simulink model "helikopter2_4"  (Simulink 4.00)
settings: Solver=ode1  SolverMode=SingleTasking  StartTime=0.0  StopTime=999999  FixedStep=0.005  MaxStep=10  RelTol=1e-3  AbsTol=1e-3
undefined symbols (not defined in the file or in its folder): simget
libraries: qctools x7

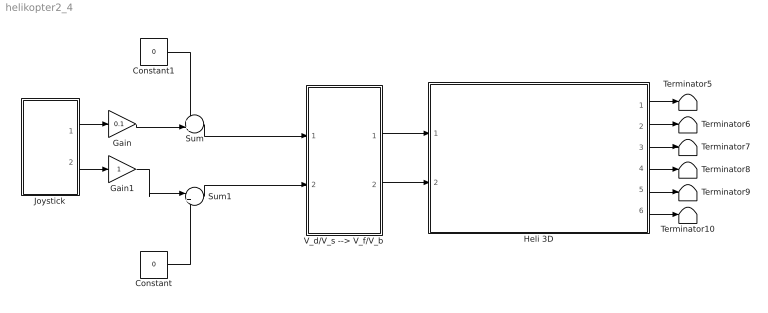
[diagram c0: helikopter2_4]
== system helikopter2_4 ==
  Constant : Constant  Value=0
  Constant1 : Constant  Value=0
  Gain : Gain  Gain=0.1  Multiplication=Element-wise(K.*u)  SaturateOnIntegerOverflow=on
  Gain1 : Gain  Gain=1  Multiplication=Element-wise(K.*u)  SaturateOnIntegerOverflow=on
  Heli 3D : Subsystem
  Joystick : Subsystem
  Sum : Sum  Inputs=++|  SaturateOnIntegerOverflow=on
  Sum1 : Sum  Inputs=|++  SaturateOnIntegerOverflow=on
  Terminator{5..10} (6 alike) : Terminator
  V_d/V_s --> V_f/V_b : Subsystem
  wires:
  V_d/V_s --> V_f/V_b/2(V_b) -> Heli 3D/2("V_b, motor bak")
  V_d/V_s --> V_f/V_b/1(V_f) -> Heli 3D/1("V_f, motor foran")
  Heli 3D/1("Vandring, (grader)") -> Terminator5/1
  Heli 3D/2("Vandringsrate, (grader/sek)") -> Terminator6/1
  Heli 3D/3("Pitch, (grader)") -> Terminator7/1
  Heli 3D/4("Pitchrate, (grader/sek)") -> Terminator8/1
  Heli 3D/5("Elevasjon, (grader)") -> Terminator9/1
  Heli 3D/6(Elevasjonsrate (grader/sek)) -> Terminator10/1
  Constant1/1 -> Sum/1
  Sum/1 -> V_d/V_s --> V_f/V_b/1(V_d)
  Constant/1 -> Sum1/2
  Sum1/1 -> V_d/V_s --> V_f/V_b/2(V_s)
  Joystick/2(Y Volt) -> Gain1/1
  Gain1/1 -> Sum1/1
  Joystick/1(X Volt) -> Gain/1
  Gain/1 -> Sum/2

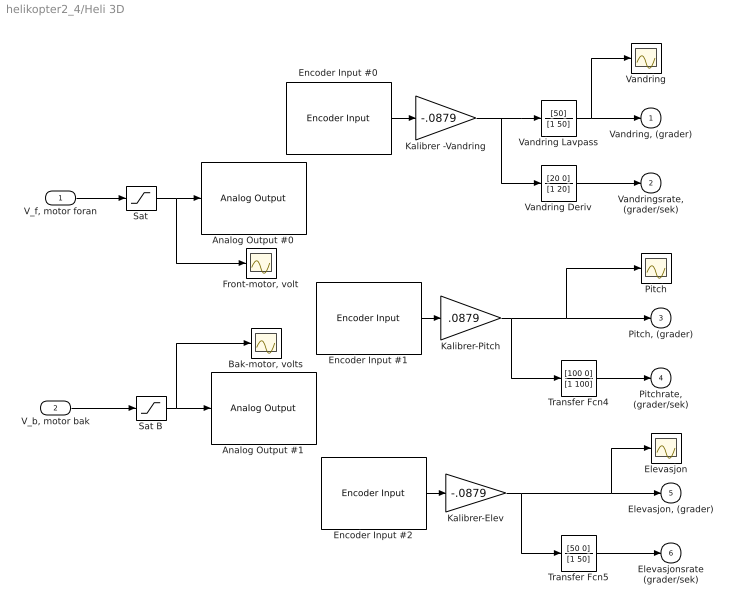
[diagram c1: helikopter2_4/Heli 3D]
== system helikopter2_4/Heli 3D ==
  "V_f, motor foran" : Inport  Port=1  LatchInput=off
  "V_b, motor bak" : Inport  Port=2  LatchInput=off
  Analog Output #0 : qctools/Quanser Consulting MQ3 Series/Analog Output  baseAddr=0x320  channels=0  initialOutputs=0  finalOutputs=0  sampleTime=-1  simulationOutput=off
  Analog Output #1 : qctools/Quanser Consulting MQ3 Series/Analog Output  baseAddr=0x320  channels=1  initialOutputs=0  finalOutputs=0  sampleTime=-1  simulationOutput=off
  "Bak-motor, volts" : Scope
  Elevasjon : Scope
  Encoder Input #0 : qctools/Quanser Consulting MQ3 Series/Encoder Input  baseAddr=0x320  channels=0  initialValues=0  sampleTime=simget(bdroot,'FixedStep')  simulationInput=off
  Encoder Input #1 : qctools/Quanser Consulting MQ3 Series/Encoder Input  baseAddr=0x320  channels=1  initialValues=0  sampleTime=simget(bdroot,'FixedStep')  simulationInput=off
  Encoder Input #2 : qctools/Quanser Consulting MQ3 Series/Encoder Input  baseAddr=0x320  channels=2  initialValues=0  sampleTime=simget(bdroot,'FixedStep')  simulationInput=off
  "Front-motor, volt" : Scope
  Kalibrer -Vandring : Gain  Gain=-.0879  Multiplication=Element-wise(K.*u)  SaturateOnIntegerOverflow=on
  Kalibrer-Elev : Gain  Gain=-.0879  Multiplication=Element-wise(K.*u)  SaturateOnIntegerOverflow=on
  Kalibrer-Pitch : Gain  Gain=.0879  Multiplication=Element-wise(K.*u)  SaturateOnIntegerOverflow=on
  Pitch : Scope
  Sat : Saturate  UpperLimit=5  LowerLimit=-5  LinearizeAsGain=on
  Sat B : Saturate  UpperLimit=5  LowerLimit=-5  LinearizeAsGain=on
  Transfer Fcn4 : TransferFcn  Numerator=[100 0]  Denominator=[1 100]  AbsoluteTolerance=auto  Realization=auto
  Transfer Fcn5 : TransferFcn  Numerator=[50 0]  Denominator=[1 50]  AbsoluteTolerance=auto  Realization=auto
  Vandring : Scope
  Vandring Deriv : TransferFcn  Numerator=[20 0]  Denominator=[1 20]  AbsoluteTolerance=auto  Realization=auto
  Vandring Lavpass : TransferFcn  Numerator=[50]  Denominator=[1 50]  AbsoluteTolerance=auto  Realization=auto
  "Vandring, (grader)" : Outport  Port=1  InitialOutput=0
  "Vandringsrate, (grader/sek)" : Outport  Port=2  InitialOutput=0
  "Pitch, (grader)" : Outport  Port=3  InitialOutput=0
  "Pitchrate, (grader/sek)" : Outport  Port=4  InitialOutput=0
  "Elevasjon, (grader)" : Outport  Port=5  InitialOutput=0
  Elevasjonsrate (grader/sek) : Outport  Port=6  InitialOutput=0
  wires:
  Vandring Deriv/1 -> "Vandringsrate, (grader/sek)"/1
  Vandring Lavpass/1 -> Vandring/1, "Vandring, (grader)"/1
  Encoder Input #0/1 -> Kalibrer -Vandring/1
  Kalibrer -Vandring/1 -> Vandring Deriv/1, Vandring Lavpass/1
  Encoder Input #1/1 -> Kalibrer-Pitch/1
  Kalibrer-Pitch/1 -> Pitch/1, "Pitch, (grader)"/1, Transfer Fcn4/1
  Transfer Fcn4/1 -> "Pitchrate, (grader/sek)"/1
  Encoder Input #2/1 -> Kalibrer-Elev/1
  Kalibrer-Elev/1 -> Transfer Fcn5/1, Elevasjon/1, "Elevasjon, (grader)"/1
  Transfer Fcn5/1 -> Elevasjonsrate (grader/sek)/1
  Sat/1 -> "Front-motor, volt"/1, Analog Output #0/1
  Sat B/1 -> "Bak-motor, volts"/1, Analog Output #1/1
  "V_f, motor foran"/1 -> Sat/1
  "V_b, motor bak"/1 -> Sat B/1

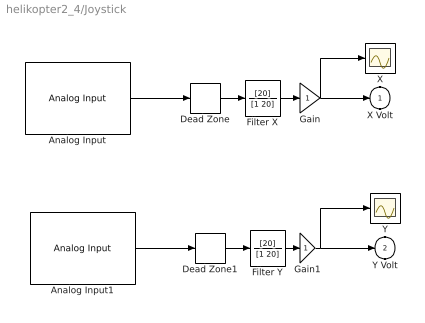
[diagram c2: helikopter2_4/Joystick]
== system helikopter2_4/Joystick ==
  Analog Input : qctools/Quanser Consulting MQ3 Series/Analog Input  baseAddr=0x320  channels=2  sampleTime=simget(bdroot,'FixedStep')  simulationInput=off
  Analog Input1 : qctools/Quanser Consulting MQ3 Series/Analog Input  baseAddr=0x320  channels=3  sampleTime=simget(bdroot,'FixedStep')  simulationInput=off
  Dead Zone : DeadZone  LowerValue=-0.5  UpperValue=0.5  SaturateOnIntegerOverflow=on  LinearizeAsGain=on
  Dead Zone1 : DeadZone  LowerValue=-0.5  UpperValue=0.5  SaturateOnIntegerOverflow=on  LinearizeAsGain=on
  Filter X : TransferFcn  Numerator=[20]  Denominator=[1 20]  AbsoluteTolerance=auto  Realization=auto
  Filter Y : TransferFcn  Numerator=[20]  Denominator=[1 20]  AbsoluteTolerance=auto  Realization=auto
  Gain : Gain  Gain=1  Multiplication=Element-wise(K.*u)  SaturateOnIntegerOverflow=on
  Gain1 : Gain  Gain=1  Multiplication=Element-wise(K.*u)  SaturateOnIntegerOverflow=on
  X : Scope
  Y : Scope
  X Volt : Outport  Port=1  InitialOutput=0
  Y Volt : Outport  Port=2  InitialOutput=0
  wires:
  Dead Zone/1 -> Filter X/1
  Analog Input1/1 -> Dead Zone1/1
  Dead Zone1/1 -> Filter Y/1
  Filter Y/1 -> Gain1/1
  Filter X/1 -> Gain/1
  Analog Input/1 -> Dead Zone/1
  Gain/1 -> X Volt/1, X/1
  Gain1/1 -> Y Volt/1, Y/1

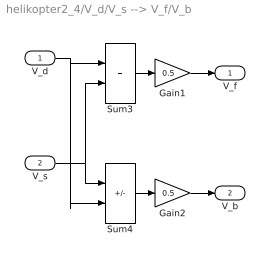
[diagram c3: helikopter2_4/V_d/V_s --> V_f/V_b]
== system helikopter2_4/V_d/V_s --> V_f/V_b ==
  V_d : Inport  Port=1  LatchInput=off
  V_s : Inport  Port=2  LatchInput=off
  Gain1 : Gain  Gain=0.5  Multiplication=Element-wise(K.*u)  SaturateOnIntegerOverflow=on
  Gain2 : Gain  Gain=0.5  Multiplication=Element-wise(K.*u)  SaturateOnIntegerOverflow=on
  Sum3 : Sum  Inputs=++  SaturateOnIntegerOverflow=on
  Sum4 : Sum  Inputs=+-  SaturateOnIntegerOverflow=on
  V_f : Outport  Port=1  InitialOutput=0
  V_b : Outport  Port=2  InitialOutput=0
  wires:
  V_s/1 -> Sum4/1, Sum3/2
  Sum3/1 -> Gain1/1
  Sum4/1 -> Gain2/1
  V_d/1 -> Sum3/1, Sum4/2
  Gain1/1 -> V_f/1
  Gain2/1 -> V_b/1
